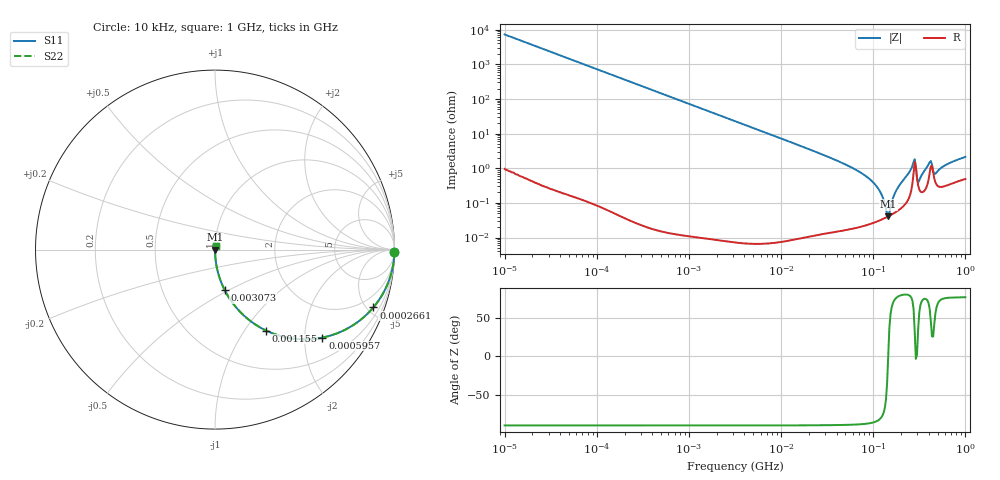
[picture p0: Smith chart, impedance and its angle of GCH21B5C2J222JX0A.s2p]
!Murata Part Number: GCH21B5C2J222JX0A
!These Parameters are Measured in Series Mode Connection
!Data Generated on Jun 19, 2026
!  o--ll--o
!Port1  Port2
!  o------o
!Operation Temp=25[degC], DC Bias Voltage=0[V]
!Freq. Start=10[kHz] Stop=1000[MHz] 401[Steps]
# Hz S RI R 50
!Freq.(Hz) S11(Real) S11(Imag) S21(Real) S21(Imag) S12(Real) S12(Imag) S22(Real) S22(Imag)
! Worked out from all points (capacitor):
!   401 points, 10 kHz to 1 GHz, reference 50 ohm
!   read as one part in series: C = 2.19 nF near 10.59 kHz
!   lowest |Z| = 40.7 mohm at 145.4 MHz (marker M1)
!   series resonance near 145.2 MHz, so ESL is about 550 pH
!   S11 on the Smith chart (normalised r, x): 10 kHz: open; 266.1 kHz: 1.00, -5.47; 595.7 kHz: 1.00, -2.44; 1.155 MHz: 1.00, -1.26; 3.073 MHz: 1.00, -0.47; 1 GHz: 1.01, +0.04
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10000  0.9998 -0.0137  0.000191 0.0137  0.000191 0.0137  0.9998 -0.0137
68786  0.9911 -0.0937  0.00886 0.0937  0.00886 0.0937  0.9911 -0.0937
266073  0.8821 -0.3224  0.1179 0.3224  0.1179 0.3224  0.8821 -0.3224
473151  0.7029 -0.4569  0.2971 0.4569  0.2971 0.4569  0.7029 -0.4569
595662  0.5989 -0.4901  0.4011 0.4901  0.4011 0.4901  0.5989 -0.4901
1154782  0.2844 -0.451  0.7156 0.451  0.7156 0.451  0.2844 -0.451
3072557  0.0532 -0.2242  0.9468 0.2242  0.9468 0.2242  0.0532 -0.2242
3162278  0.0503 -0.2185  0.9497 0.2185  0.9497 0.2185  0.0503 -0.2185
2.175204e7  0.00118 -0.0327  0.9988 0.0327  0.9988 0.0327  0.00118 -0.0327
5.463866e7  0.000302 -0.0115  0.9997 0.0115  0.9997 0.0115  0.000302 -0.0115
8.912509e7  0.000264 -0.00515  0.9997 0.00515  0.9997 0.00515  0.000264 -0.00515
1.154782e8  0.000311 -0.00237  0.9997 0.00237  0.9997 0.00237  0.000311 -0.00237
1.372461e8  0.000377 -0.000586  0.9996 0.000586  0.9996 0.000586  0.000377 -0.000586
1.453784e8  0.000407 1.27e-05  0.9996 -1.27e-05  0.9996 -1.27e-05  0.000407 1.27e-05
1.496236e8  0.000424 0.000315  0.9996 -0.000315  0.9996 -0.000315  0.000424 0.000315
1.778279e8  0.00056 0.00221  0.9994 -0.00221  0.9994 -0.00221  0.00056 0.00221
2.73842e8  0.00724 0.013  0.9928 -0.013  0.9928 -0.013  0.00724 0.013
3.162278e8  0.00243 0.00375  0.9976 -0.00375  0.9976 -0.00375  0.00243 0.00375
4.097321e8  0.00724 0.0129  0.9928 -0.0129  0.9928 -0.0129  0.00724 0.0129
4.869675e8  0.00338 0.0068  0.9966 -0.0068  0.9966 -0.0068  0.00338 0.0068
6.309573e8  0.00334 0.0125  0.9967 -0.0125  0.9967 -0.0125  0.00334 0.0125
1e9  0.00529 0.0205  0.9947 -0.0205  0.9947 -0.0205  0.00529 0.0205
